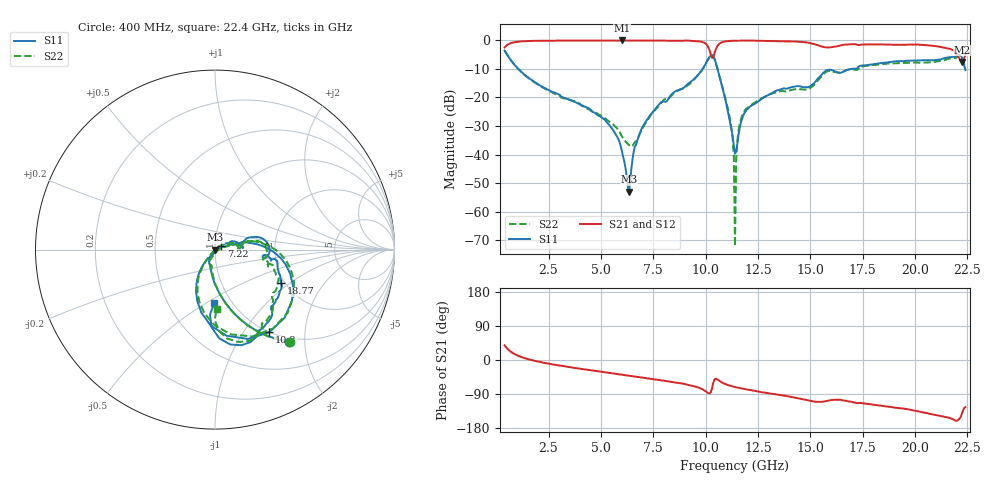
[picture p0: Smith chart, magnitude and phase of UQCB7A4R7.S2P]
!  Part Number  UQCB7A4R7	Mounting Orientation: Vertical
!  Description: RF capacitors
!  Application: Coupling, Bypass, Tuning, DC Block
!  Filters, Matching
# GHZ S DB R 50
! Freq  |S11|  S11 Ph  |S21|  S21 Ph  |S12|  S12 Ph  |S22|  S22 Ph
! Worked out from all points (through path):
!   401 points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, 400 MHz to 22.4 GHz, reference 50 ohm
!   highest |S21| = -0.09 dB at 6.01 GHz (marker M1); lowest = -7.6 dB at 22.23 GHz (marker M2)
!   group delay of S21, straight-line fit = 20.1 ps
!   lowest |S11| = -53.0 dB at 6.34 GHz (marker M3), VSWR 1.00, Z = 50.2 - j0.107 ohm
!   |S11| at or under -10 dB: 1.047 GHz to 9.859 GHz (8.812 GHz wide, 162 % of centre); 10.56 GHz to 16.98 GHz (6.421 GHz wide, 46.6 % of centre); 22.38438 GHz to end of sweep
!   |S22| runs from -72.1 to -3.6 dB; largest |S21 - S12| = 0.0046
!   S11 on the Smith chart (normalised r, x): 400 MHz: 0.93, -1.69; 7.22 GHz: 1.07, +0.05; 10.3 GHz: 1.00, -1.32; 18.77 GHz: 1.91, -0.86; 22.4 GHz: 0.83, -0.54
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0.4  -3.62 -51.0  -2.54 38.5  -2.54 38.5  -3.60 -51.0
1.335  -11.98 -83.5  -0.36 5.2  -0.36 5.2  -12.04 -83.6
4.085  -22.76 -116.6  -0.16 -23.5  -0.16 -23.5  -22.92 -115.5
5.295  -28.81 -128.2  -0.13 -33.3  -0.13 -33.3  -27.95 -109.2
6.01  -39.16 -127.2  -0.09 -38.8  -0.09 -38.8  -33.78 -90.5
6.34  -52.98 -28.4  -0.10 -41.4  -0.10 -41.4  -36.65 -58.0
6.67  -36.63 30.6  -0.11 -44.0  -0.10 -44.0  -35.54 -13.9
7.22  -27.64 33.3  -0.12 -48.4  -0.12 -48.4  -28.12 14.6
7.77  -22.48 28.1  -0.16 -52.9  -0.15 -52.9  -22.86 16.1
9.805  -10.58 1.1  -0.57 -76.1  -0.56 -76.1  -10.69 4.7
10.3  -5.18 -56.6  -6.14 -75.4  -6.14 -75.5  -5.26 -53.4
10.575  -10.36 -109.0  -1.85 -52.0  -1.85 -52.1  -10.32 -106.5
11.07  -25.38 -125.7  -0.32 -66.3  -0.31 -66.3  -24.22 -130.3
11.4  -39.72 -57.2  -0.17 -71.5  -0.16 -71.5  -72.06 -17.6
11.51  -36.23 4.0  -0.17 -72.9  -0.17 -73.0  -35.44 38.2
11.62  -30.88 20.1  -0.17 -74.1  -0.17 -74.1  -29.55 35.5
11.95  -24.43 16.6  -0.12 -77.7  -0.11 -77.8  -23.90 22.9
15.085  -15.61 15.9  -1.17 -108.7  -1.17 -108.8  -16.25 9.4
18.77  -7.69 -27.0  -1.54 -123.9  -1.50 -123.9  -8.14 -25.2
21.245  -6.65 -47.0  -2.40 -148.3  -2.40 -148.6  -7.19 -42.9
22.235  -6.10 -87.2  -7.59 -141.7  -7.58 -141.9  -6.01 -82.1
22.4  -10.48 -91.0  -5.10 -124.5  -5.09 -124.7  -9.55 -88.4
